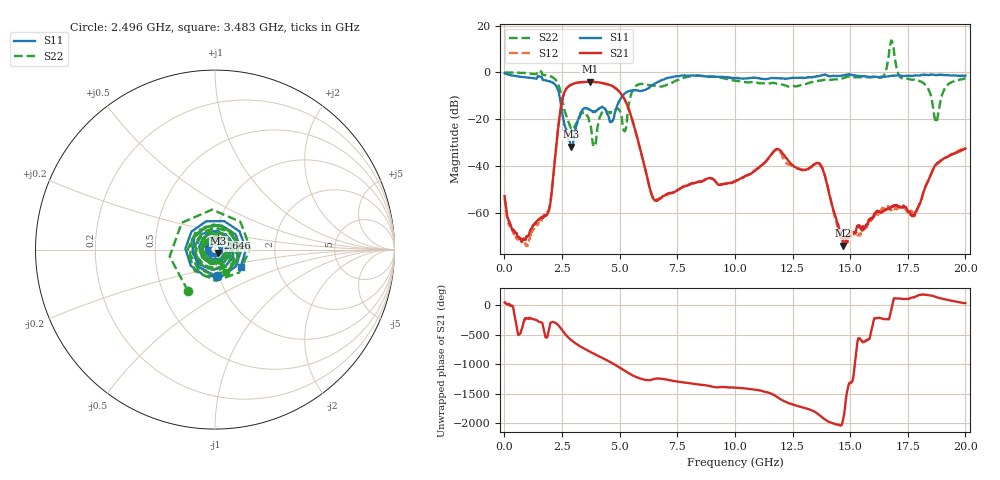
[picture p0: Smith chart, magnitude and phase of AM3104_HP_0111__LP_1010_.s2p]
!Created with skrf (http://scikit-rf.org).
# Hz S RI R 50.0
!freq ReS11 ImS11 ReS21 ImS21 ReS12 ImS12 ReS22 ImS22
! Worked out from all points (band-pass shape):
!   1601 points, 10 MHz to 20 GHz, reference 50 ohm
!   highest |S21| = -3.97 dB at 3.708 GHz (marker M1); lowest = -74.1 dB at 14.7 GHz (marker M2)
!   |S21| within 3 dB of the highest: 2.69 GHz to 4.854 GHz (2.164 GHz wide, 57.4 % of centre)
!   lowest |S11| = -31.7 dB at 2.884 GHz (marker M3), VSWR 1.05, Z = 51.8 - j1.92 ohm
!   |S11| at or under -10 dB: 2.39 GHz to 5.13 GHz (2.74 GHz wide, 72.9 % of centre)
!   |S22| runs from -31.4 to 13.6 dB; largest |S21 - S12| = 0.051
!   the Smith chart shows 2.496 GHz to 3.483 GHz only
!   S11 on the Smith chart (normalised r, x): 2.496 GHz: 0.97, -0.30; 2.646 GHz: 1.02, +0.14; 3.483 GHz: 1.30, -0.26
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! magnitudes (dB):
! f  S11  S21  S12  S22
! 10 MHz  -0.4  -52.9  -53.6  0.0
! 934.5 MHz  -2.1  -71.3  -73.4  -0.3
! 1.847 GHz  -3.5  -60.9  -60.0  -1.2
! 2.496 GHz  -16.5  -12.4  -12.4  -11.2
! 2.646 GHz  -23.4  -7.7  -7.6  -17.4
! 2.884 GHz  -31.7  -5.3  -5.4  -23.8
! 3.346 GHz  -16.7  -4.2  -4.3  -17.4
! 3.483 GHz  -15.2  -4.1  -4.1  -17.0
! 3.708 GHz  -15.9  -4.0  -4.0  -21.8
! 4.658 GHz  -21.0  -5.7  -5.9  -16.9
! 5.17 GHz  -9.5  -10.7  -10.7  -24.6
! 5.682 GHz  -7.6  -24.9  -24.9  -6.1
! 6.682 GHz  -4.0  -54.4  -54.2  -6.0
! 10.01 GHz  -2.5  -46.6  -46.7  -3.6
! 11.83 GHz  -2.5  -32.8  -32.9  -4.9
! 13.34 GHz  -2.1  -40.1  -40.1  -4.2
! 13.79 GHz  -1.1  -40.8  -40.6  -3.3
! 14.7 GHz  -1.3  -74.1  -72.2  -2.5
! 16.68 GHz  -1.6  -58.2  -57.5  7.3
! 17.78 GHz  -1.3  -61.3  -60.7  -3.1
! 18.73 GHz  -1.2  -39.3  -39.5  -21.4
! 20 GHz  -1.4  -32.5  -32.0  -2.6
